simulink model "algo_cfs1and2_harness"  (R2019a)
settings: configuration reference "configurationSettings" (kept in a data dictionary, not in this file)
undefined symbols (not defined in the file or in its folder): algo_cfs1_fp, algo_cfs2_fp

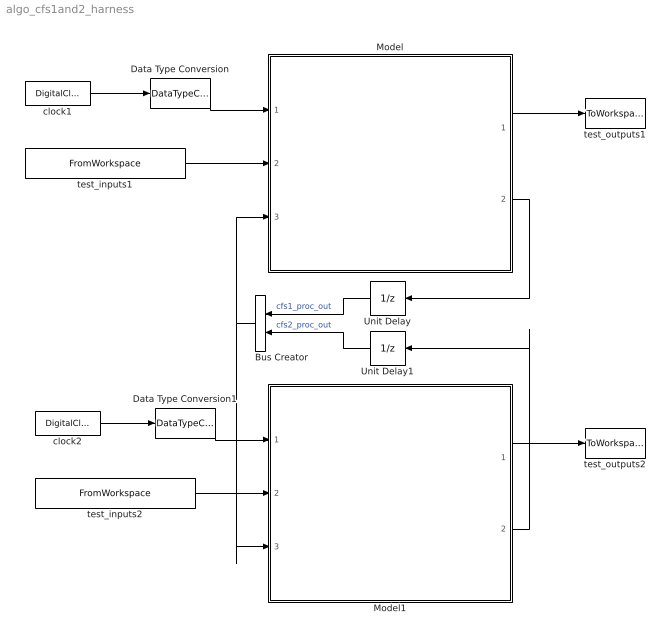
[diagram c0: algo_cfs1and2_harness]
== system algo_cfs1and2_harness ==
  Bus Creator : BusCreator  Inputs=2
  Data Type Conversion : DataTypeConversion  OutDataTypeStr=single
  Data Type Conversion1 : DataTypeConversion  OutDataTypeStr=single
  Model : ModelReference  ModelNameDialog=algo_cfs1.slx  SimulationMode=Normal  ModelReferenceVersion=1.793  SimulationMode=Normal
  Model1 : ModelReference  ModelNameDialog=algo_cfs2.slx  SimulationMode=Normal  ModelReferenceVersion=1.790  SimulationMode=Normal
  Unit Delay : UnitDelay  SampleTime=-1  HasFrameUpgradeWarning=on
  Unit Delay1 : UnitDelay  SampleTime=-1  HasFrameUpgradeWarning=on
  clock1 : DigitalClock  SampleTime=algo_cfs1_fp.timing.dt
  clock2 : DigitalClock  SampleTime=algo_cfs1_fp.timing.dt
  test_inputs1 : FromWorkspace  VariableName=algo_cfs1_inbus1  OutDataTypeStr=Bus: algo_cfs1_inBus  SampleTime=algo_cfs1_fp.timing.dt  Interpolate=off  OutputAfterFinalValue=Holding final value
  test_inputs2 : FromWorkspace  VariableName=algo_cfs2_inbus1  OutDataTypeStr=Bus: algo_cfs2_inBus  SampleTime=algo_cfs2_fp.timing.dt  Interpolate=off  OutputAfterFinalValue=Holding final value
  test_outputs1 : ToWorkspace  VariableName=simout1  SaveFormat=Timeseries  SampleTime=-1
  test_outputs2 : ToWorkspace  VariableName=simout2  SaveFormat=Timeseries  SampleTime=-1
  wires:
  Model/1 -> test_outputs1/1
  clock1/1 -> Data Type Conversion/1
  Data Type Conversion/1 -> Model/1
  Model1/1 -> test_outputs2/1
  Data Type Conversion1/1 -> Model1/1
  clock2/1 -> Data Type Conversion1/1
  test_inputs1/1 -> Model/2
  test_inputs2/1 -> Model1/2
  Model/2 -> Unit Delay/1
  Model1/2 -> Unit Delay1/1
  Unit Delay/1 -> Bus Creator/1  "cfs1_proc_out"
  Unit Delay1/1 -> Bus Creator/2  "cfs2_proc_out"
  Bus Creator/1 -> Model/3, Model1/3
